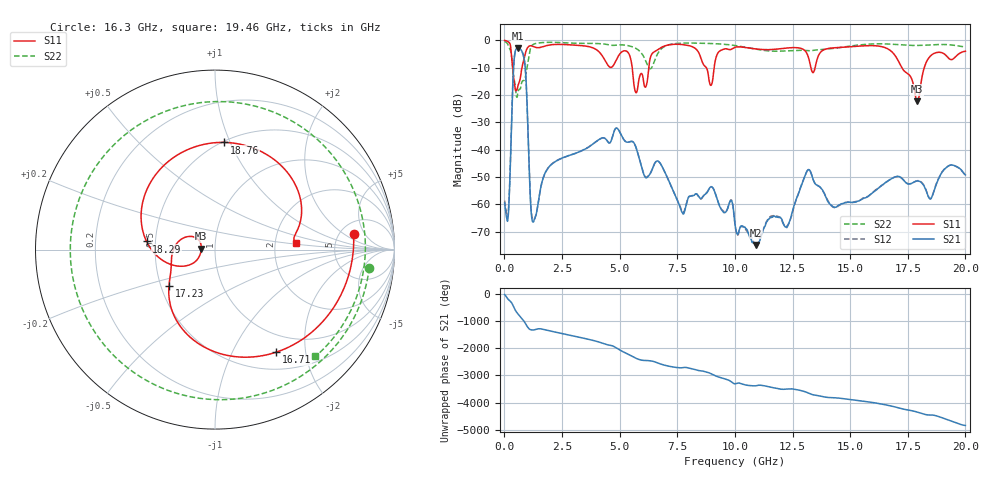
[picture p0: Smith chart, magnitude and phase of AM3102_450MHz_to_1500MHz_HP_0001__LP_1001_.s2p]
!Agilent Technologies,E8364B,MY43040894,A.07.50.67
!Agilent E8364B: A.07.50.67
!Date: Thursday, January 11, 2018 05:21:45
!Correction: S11(Full 2 Port(1,2))
!S21(Full 2 Port(1,2))
!S12(Full 2 Port(1,2))
!S22(Full 2 Port(1,2))
!S2P File: Measurements: S11, S21, S12, S22:
# Hz S  dB  R 50
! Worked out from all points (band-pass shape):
!   1601 points, 10 MHz to 20 GHz, reference 50 ohm
!   highest |S21| = -2.93 dB at 584.7 MHz (marker M1); lowest = -74.9 dB at 10.93 GHz (marker M2)
!   |S21| within 3 dB of the highest: 436.4 MHz to 835.8 MHz (399.4 MHz wide, 62.8 % of centre)
!   lowest |S11| = -22.3 dB at 17.91 GHz (marker M3), VSWR 1.17, Z = 42.9 + j0.457 ohm
!   |S11| at or under -10 dB: 356.1 MHz to 762.5 MHz (406.5 MHz wide, 72.7 % of centre); 5.545 GHz to 6.262 GHz (717.5 MHz wide, 12.2 % of centre); 17.24 GHz to 18.22 GHz (971.7 MHz wide, 5.48 % of centre)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
!   |S22| runs from -20.9 to -0.4 dB; largest |S21 - S12| = 0.0023
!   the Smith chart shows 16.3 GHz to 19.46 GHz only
!   S11 on the Smith chart (normalised r, x): 16.3 GHz: 6.63, +2.97; 16.71 GHz: 0.73, -1.50; 17.23 GHz: 0.55, -0.25; 18.29 GHz: 0.45, +0.05; 18.76 GHz: 0.51, +0.95; 19.46 GHz: 2.64, +0.23
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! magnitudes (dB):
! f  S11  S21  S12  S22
! 10 MHz  0.0  -59.5  -58.6  -0.4
! 159.9 MHz  -0.5  -64.8  -63.9  -1.6
! 409.8 MHz  -14.3  -8.6  -8.6  -13.5
! 584.7 MHz  -16.8  -2.9  -2.9  -19.0
! 884.6 MHz  -5.7  -8.3  -8.3  -14.4
! 1.259 GHz  -2.3  -66.5  -65.5  -1.5
! 3.346 GHz  -1.9  -40.4  -40.5  -1.1
! 5.707 GHz  -19.2  -39.1  -39.1  -3.0
! 6.682 GHz  -3.3  -44.3  -44.3  -4.4
! 8.956 GHz  -16.5  -53.6  -53.6  -1.2
! 10.01 GHz  -2.5  -67.3  -67.6  -1.9
! 10.93 GHz  -3.2  -74.9  -75.3  -3.2
! 13.34 GHz  -11.3  -49.5  -49.5  -3.7
! 16.3 GHz  -2.2  -53.5  -53.6  -1.3
! 16.68 GHz  -3.3  -51.2  -51.2  -1.4
! 16.71 GHz  -3.5  -51.1  -51.0  -1.4
! 17.23 GHz  -9.7  -50.4  -50.4  -1.7
! 17.91 GHz  -22.3  -51.4  -51.4  -1.9
! 18.29 GHz  -8.3  -54.8  -54.7  -1.8
! 18.76 GHz  -4.4  -52.1  -52.0  -1.6
! 19.46 GHz  -6.8  -45.7  -45.7  -1.8
! 20 GHz  -4.0  -49.3  -49.2  -2.4
